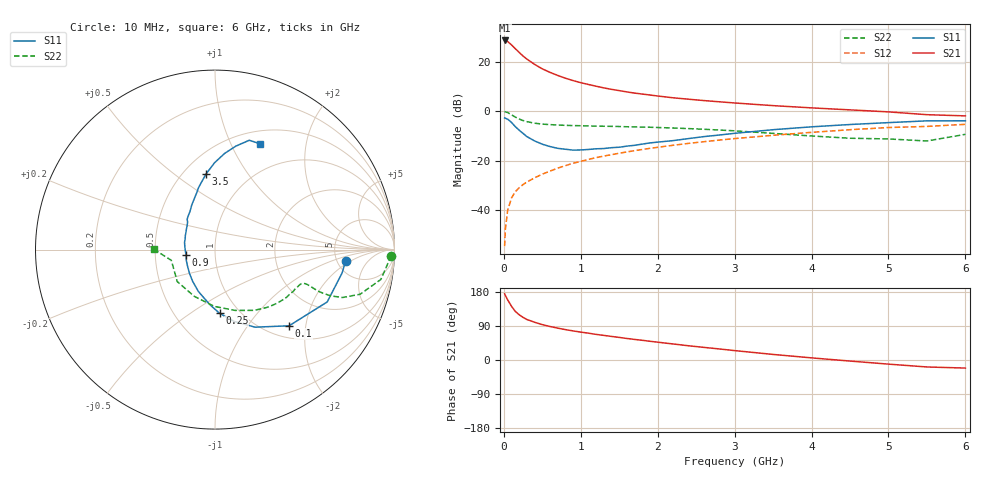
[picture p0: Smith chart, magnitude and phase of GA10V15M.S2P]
! Infineon Technologies  Discrete & RF Semiconductors
! BF775
! Si NPN RF Bipolar Junction Transistor in SOT23
! VCE = 10 V  IC = 15 mA
! Common Emitter S-Parameters:  May  1996
# GHz  S  MA  R  50
!  f  S11  S21  S12  S22
! GHz  MAG  ANG  MAG  ANG  MAG  ANG  MAG  ANG
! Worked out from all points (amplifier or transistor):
!   36 points, 10 MHz to 6 GHz, reference 50 ohm
!   highest |S21| = 28.5 dB at 10 MHz (marker M1)
!   |S21| within 3 dB of that: start of sweep to 139.3 MHz
!   unconditionally stable (mu >= 1): 527.9 MHz to 2.68 GHz
!   at 250 MHz: K = 0.75, MSG = 25.9 dB, |S12| = -29.6 dB
!   at 1.4 GHz: K = 1.09, MAG = 11.3 dB, |S12| = -17.5 dB
!   at 6 GHz: K = 0.88, MSG = 1.7 dB, |S12| = -5.3 dB
!   S11 on the Smith chart (normalised r, x): 10 MHz: 5.96, -1.62; 100 MHz: 1.24, -1.62; 250 MHz: 0.81, -0.66; 900 MHz: 0.72, -0.05; 3.5 GHz: 0.64, +0.66; 6 GHz: 0.65, +1.29
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0.01  0.7302 -5.0  26.65 174.8  0.0019 85.9  0.9835 -2.0
0.02  0.7201 -10.4  26.5 170.4  0.0042 80.3  0.9683 -4.2
0.05  0.6899 -25.0  25.31 158.5  0.0101 79.1  0.939 -10.2
0.1  0.5921 -45.8  21.7 141.6  0.0178 70.8  0.8459 -17.1
0.15  0.4864 -62.7  18.16 128.0  0.0239 66.4  0.7587 -20.6
0.2  0.4134 -75.2  15.27 119.3  0.0287 65.6  0.6938 -21.8
0.25  0.3559 -85.9  12.93 112.4  0.0332 65.0  0.6471 -22.0
0.3  0.3073 -95.5  11.22 106.9  0.0374 65.6  0.6145 -21.9
0.4  0.2511 -111.6  8.78 99.6  0.0453 66.9  0.573 -21.1
0.5  0.2159 -125.3  7.134 93.3  0.0538 67.7  0.5486 -20.7
0.6  0.1937 -137.5  6.058 88.4  0.0619 68.3  0.5359 -20.7
0.7  0.1783 -149.2  5.257 84.1  0.071 68.6  0.5262 -21.0
0.8  0.1709 -159.1  4.623 80.2  0.0798 68.5  0.518 -21.5
0.9  0.1641 -169.0  4.137 76.8  0.0891 68.5  0.5127 -22.2
1.1  0.1691 173.9  3.45 70.8  0.1066 68.1  0.5046 -24.3
1.3  0.1765 160.3  2.947 64.9  0.1245 66.8  0.4968 -26.5
1.6  0.1975 143.5  2.443 56.8  0.151 65.0  0.4854 -30.6
2.2  0.255 123.0  1.862 42.3  0.2055 60.0  0.4584 -40.4
3.5  0.4233 96.9  1.294 14.7  0.3268 46.4  0.3568 -71.7
4.5  0.5386 84.3  1.063 -2.8  0.4231 34.2  0.2849 -113.9
5.5  0.6384 72.6  0.85 -18.4  0.4931 19.0  0.2507 -166.2
6  0.6406 67.2  0.804 -21.3  0.5432 14.8  0.3414 179.6
